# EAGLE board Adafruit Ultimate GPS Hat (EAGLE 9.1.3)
REV: B
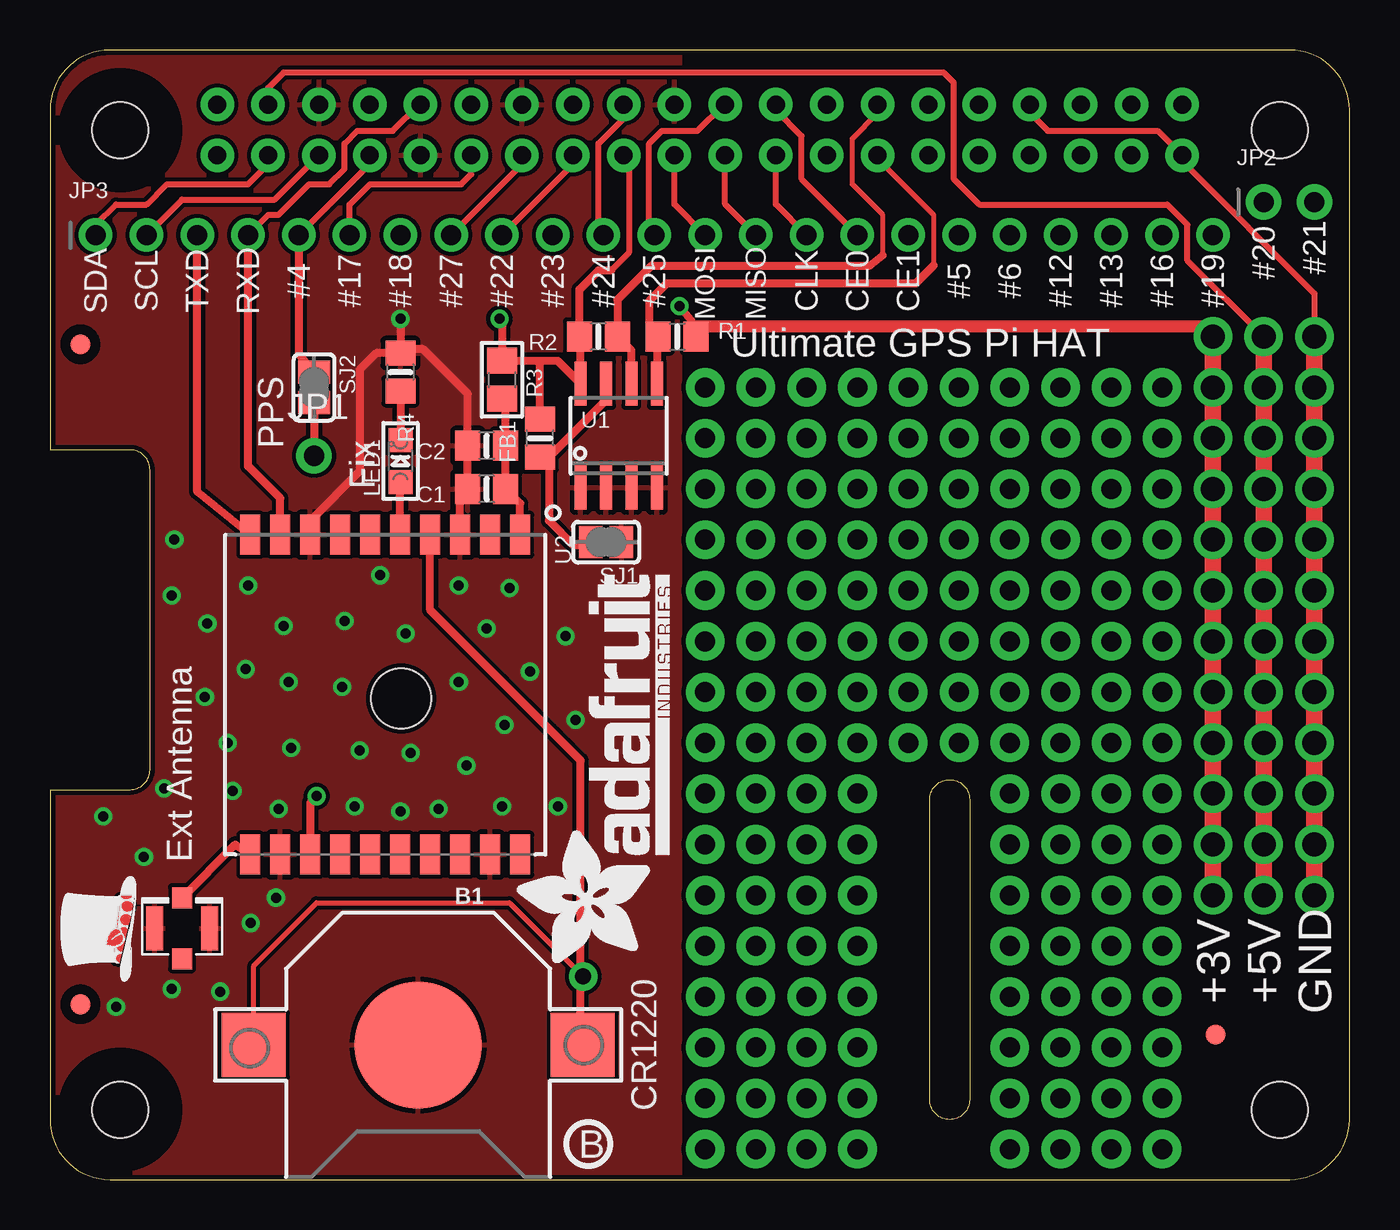
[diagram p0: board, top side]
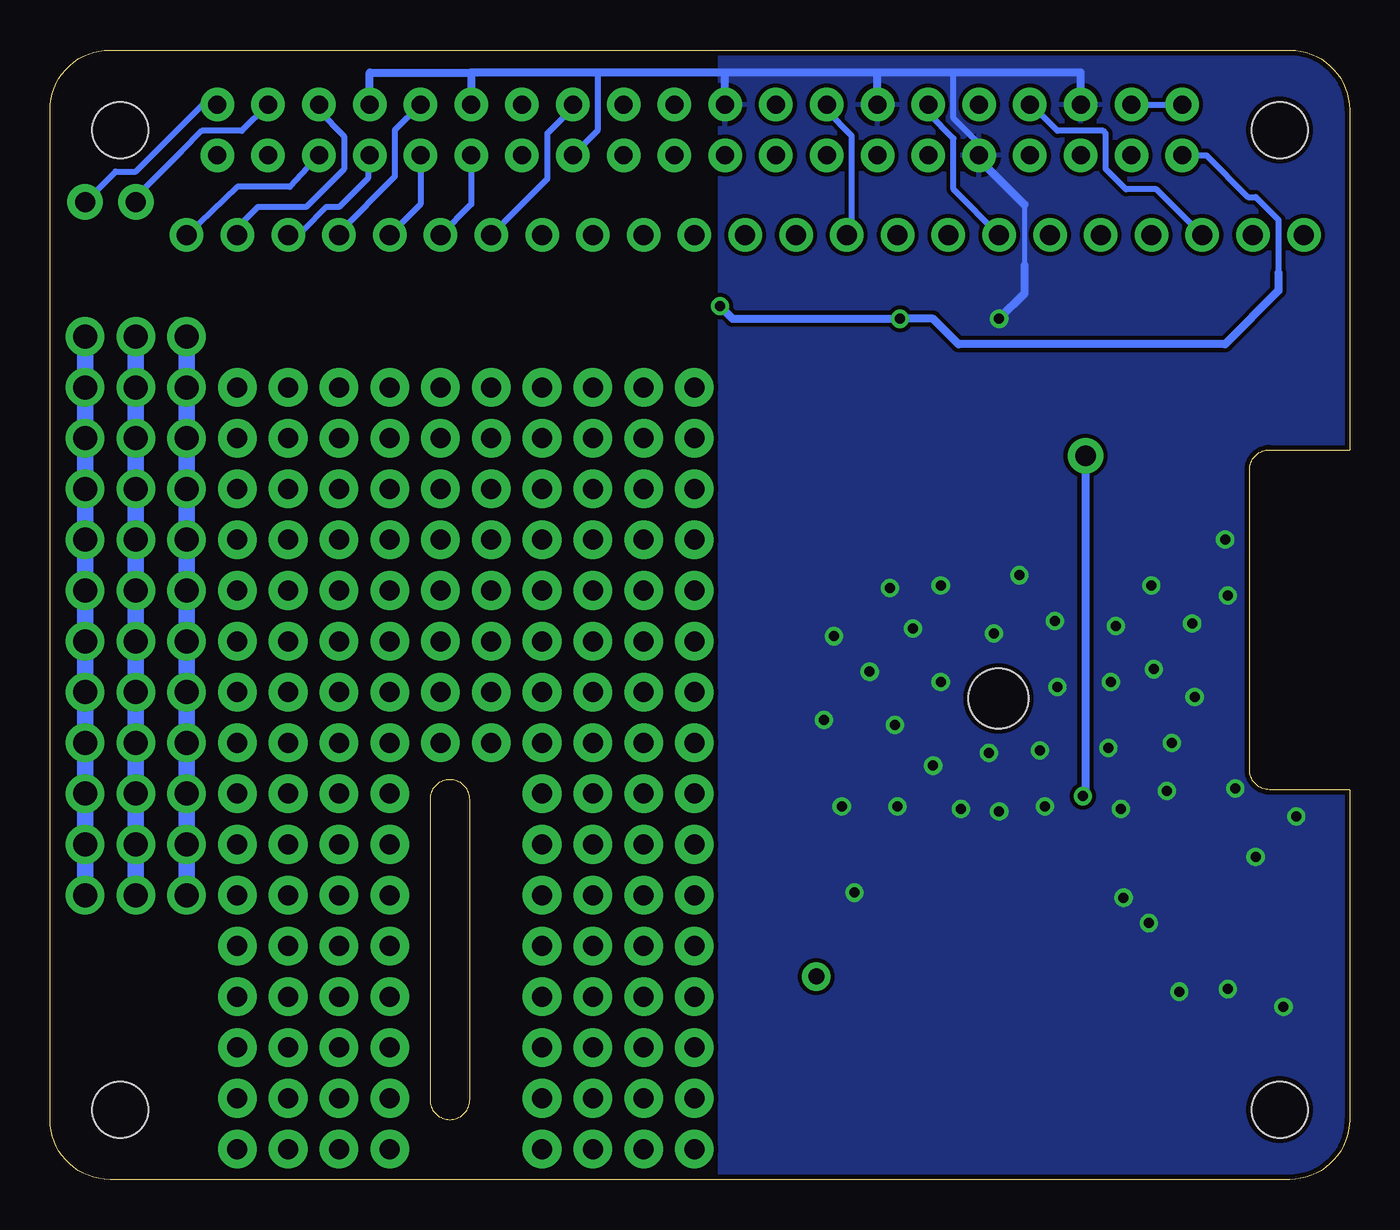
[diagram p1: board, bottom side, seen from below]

Size 65 x 56.5 mm. Coordinates in mm from the lower left corner, seen from the top.
Copper layers (1*16): Top 0.035mm / dielectric 1.5mm / Bottom 0.035mm
Design rules "adafruit": minimum track width 8mil, minimum drill 15.5mil, track to track 8mil, track to pad 8mil, pad to pad 8mil, via to via 8mil, smd to smd 8mil, copper to edge 10mil, drill to drill 8mil, minimum pad ring 10mil, minimum via ring 8mil, stop-mask expansion 2mil, vias tented up to drill 20mil, thermal gap 10mil

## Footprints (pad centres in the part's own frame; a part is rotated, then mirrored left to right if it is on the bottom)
CR1220 = smd 3.2 x 3.2: +$1 -8.225,0; +$2 8.225,0 | smd 6.35 x 6.35: - 0,0
0805-NO = smd 1.24 x 1.5: 1 -0.95,0; 2 0.95,0
0805 = smd 1.3 x 1.5: 1 -0.95,0; 2 0.95,0
FIDUCIAL_1MM = smd 1 x 1: 1 0,0
1X01-CLEANBIG = drill 1.016 pad 1.778: 1 0,0
1X02_ROUND = drill 1 pad 1.778: 1 -1.27,0; 2 1.27,0
1X23_ROUND_70MIL = drill 1 pad 1.676: 1 -27.94,0; 2 -25.4,0; 3 -22.86,0; 4 -20.32,0; 5 -17.78,0; 6 -15.24,0; 7 -12.7,0; 8 -10.16,0; 9 -7.62,0; 10 -5.08,0; 11 -2.54,0; 12 0,0; 13 2.54,0; 14 5.08,0; 15 7.62,0; 16 10.16,0; 17 12.7,0; 18 15.24,0; 19 17.78,0; 20 20.32,0; 21 22.86,0; 22 25.4,0; 23 27.94,0
CHIPLED_0805 = smd 1.2 x 1.2: A 0,-1.05; C 0,1.05
PI_HAT_SLOTS = drill 0.9 pad 1.676: 1 8.37,51.23; 2 8.37,53.77; 3 10.91,51.23; 4 10.91,53.77; 5 13.45,51.23; 6 13.45,53.77; 7 15.99,51.23; 8 15.99,53.77; 9 18.53,51.23; 10 18.53,53.77; 11 21.07,51.23; 12 21.07,53.77; 13 23.61,51.23; 14 23.61,53.77; 15 26.15,51.23; 16 26.15,53.77; 17 28.69,51.23; 18 28.69,53.77; 19 31.23,51.23; 20 31.23,53.77; 21 33.77,51.23; 22 33.77,53.77; 23 36.31,51.23; 24 36.31,53.77; 25 38.85,51.23; 26 38.85,53.77; 27 41.39,51.23; 28 41.39,53.77; 29 43.93,51.23; 30 43.93,53.77; 31 46.47,51.23; 32 46.47,53.77; 33 49.01,51.23; 34 49.01,53.77; 35 51.55,51.23; 36 51.55,53.77; 37 54.09,51.23; 38 54.09,53.77; 39 56.63,51.23; 40 56.63,53.77 | hole 2.8: 3.5,3.5; 3.5,52.5; 61.5,52.5; 61.5,3.5
SOLDERJUMPER_CLOSEDWIRE = smd 1.168 x 1.6: 1 -0.762,0; 2 0.762,0 | smd 0.635 x 0.203: WIRE 0,0
SOIC8_150MIL = smd 0.6 x 2.2: 1 -1.905,-2.6; 2 -0.635,-2.6; 3 0.635,-2.6; 4 1.905,-2.6; 5 1.905,2.6; 6 0.635,2.6; 7 -0.635,2.6; 8 -1.905,2.6
FGPMMOPA6H = smd 2 x 1: P$1 -8,6.75; P$2 -8,5.25; P$3 -8,3.75; P$4 -8,2.25; P$5 -8,0.75; P$6 -8,-0.75; P$7 -8,-2.25; P$8 -8,-3.75; P$9 -8,-5.25; P$10 -8,-6.75; P$11 8,-6.75; P$12 8,-5.25; P$13 8,-3.75; P$14 8,-2.25; P$15 8,-0.75; P$16 8,0.75; P$17 8,2.25; P$18 8,3.75; P$19 8,5.25; P$20 8,6.75 | hole 3: 0.2,0.8
U.FL = smd 2.2 x 0.85: P$1 0,1.375; P$2 0,-1.375 | smd 1.05 x 1: P$3 1.525,0; P$4 -1.525,0

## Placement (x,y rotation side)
B1  CR1220  [CR1220]  18.41,6.73 180 top
C1  0.1uF  [0805-NO]  21.84,34.54 180 top
C2  10uF  [0805-NO]  21.84,36.7 180 top
FB1  Ferrite  [0805]  22.61,40.01 270 top
FID1  FIDUCIAL_1MM  [FIDUCIAL_1MM]  1.52,8.76 0 top
FID2  FIDUCIAL_1MM  [FIDUCIAL_1MM]  1.52,41.78 0 top
FID3  FIDUCIAL_1MM  [FIDUCIAL_1MM]  58.29,7.24 0 top
JP1  [1X01-CLEANBIG]  13.21,36.2 0 top
JP2  [1X02_ROUND]  61.98,48.9 0 top
JP3  [1X23_ROUND_70MIL]  30.23,47.24 0 top
LED1  RED  [CHIPLED_0805]  17.53,35.94 0 top
R1  3.9K  [0805-NO]  31.37,42.16 0 top
R2  3.9K  [0805-NO]  27.43,42.16 180 top
R3  3.9K  [0805-NO]  24.51,37.08 90 top
R4  470  [0805-NO]  17.53,40.39 270 top
RPI1  RASPBERRYPI_BPLUS_HATSLOTS  [PI_HAT_SLOTS]  0,0 0 top
SJ1  WP  [SOLDERJUMPER_CLOSEDWIRE]  27.81,31.88 180 top
SJ2  PPS  [SOLDERJUMPER_CLOSEDWIRE]  13.21,39.62 270 top
U1  CAT24C32  [SOIC8_150MIL]  28.45,37.21 0 top
U2  FGPMMOPA6H  [FGPMMOPA6H]  16.76,24.26 270 top
U$3  [ADAFRUIT_TEXT_20MM]  30.99,10.67 90 top
U$4  [PIHATLOGO]  4.32,9.91 90 top
U$6  [PCBFEAT-REV-056]  26.92,1.78 0 top
U$20  U.FL  [U.FL]  6.6,12.57 90 top

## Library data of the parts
B1 C1 C2 FB1 JP2 JP3 LED1 R1-R4 RPI1 SJ1 SJ2 U1 U2 U$3 U$4 U$6 U$20 = microbuilder
FID1-FID3 = microbuilder; BOM: EXCLUDE
JP1 = adafruit

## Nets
1PPS: JP1.1 SJ2.2 U2.P$13
3.3V: FB1.1 R1.2 R2.2 R3.2 RPI1.1 RPI1.17 U1.8
5.0V: RPI1.2 RPI1.4
EECLK: R2.1 RPI1.28 U1.6
EEDATA: R1.1 RPI1.27 U1.5
FIX: LED1.A U2.P$5
GND: B1.- C1.2 C2.2 R4.1 RPI1.6 RPI1.9 RPI1.14 RPI1.20 RPI1.25 RPI1.30 RPI1.34 RPI1.39 SJ1.1 U1.1 U1.2 U1.3 U1.4 U2.P$3 U2.P$8 U2.P$12 U2.P$19 U$20.P$1 U$20.P$2
GPIO4: JP3.5 RPI1.7 SJ2.1
GPIO5: JP3.18 RPI1.29
GPIO6: JP3.19 RPI1.31
GPIO12: JP3.20 RPI1.32
GPIO13: JP3.21 RPI1.33
GPIO16: JP3.22 RPI1.36
GPIO17: JP3.6 RPI1.11
GPIO18: JP3.7 RPI1.12
GPIO19: JP3.23 RPI1.35
GPIO20: JP2.1 RPI1.38
GPIO21: JP2.2 RPI1.40
GPIO22: JP3.9 RPI1.15
GPIO23: JP3.10 RPI1.16
GPIO24: JP3.11 RPI1.18
GPIO25: JP3.12 RPI1.22
GPIO26: RPI1.37
GPIO27: JP3.8 RPI1.13
N$16: R3.1 SJ1.2 U1.7
N$24: LED1.C R4.2
N$26: U2.P$11 U$20.P$3
RXD: JP3.4 RPI1.10 U2.P$9
SCL: JP3.2 RPI1.5
SDA: JP3.1 RPI1.3
SPI_CE0: JP3.16 RPI1.24
SPI_CE1: JP3.17 RPI1.26
SPI_MISO: JP3.14 RPI1.21
SPI_MOSI: JP3.13 RPI1.19
SPI_SCLK: JP3.15 RPI1.23
TXD: JP3.3 RPI1.8 U2.P$10
VBACKUP: B1.+$1 B1.+$2 U2.P$4
VCC: C1.1 C2.1 FB1.2 U2.P$1

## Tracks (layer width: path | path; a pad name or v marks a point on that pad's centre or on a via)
1PPS  (via drill 0.5)
  Top 0.406: SJ2.2 JP1.1 | v13.34,19.18 13.01,18.86 U2.P$13
  Bottom 0.406: JP1.1 13.21,19.3 v13.34,19.18
3.3V  (via drill 0.5, 1.2 pad 1.93)
  Top 0.305: RPI1.17 28.96,50.96 28.96,46.36 28.07,45.47
  Top 0.406: 24.64,40.95 FB1.1 22.61,42.93 v22.48,43.05 | 24.64,40.95 25.4,40.95 U1.8 26.54,42.23 R2.2 26.48,44.52 27.43,45.47 28.07,45.47 | R1.2 32.07,42.99 v31.5,43.69 | R3.2 24.51,40.83 24.64,40.95
  Top 0.61: v58.17,42.16 57.66,42.67 32,42.67 32.07,42.61 R1.2
  Top 0.813: v58.17,42.16 v58.17,14.22
  Bottom 0.305: RPI1.1 7.16,51.23 5.08,49.15 4.7,49.15 3.56,48.01 3.56,45.34
  Bottom 0.406: 3.56,45.34 3.56,44.45 6.22,41.78 19.56,41.78 20.83,43.05 v22.48,43.05 30.86,43.05 v31.5,43.69
  Bottom 0.813: v58.17,14.22 v58.17,16.76 v58.17,19.3 v58.17,21.84 v58.17,24.38 v58.17,26.92 v58.17,29.46 v58.17,32 v58.17,34.54 v58.17,37.08 v58.17,39.62 v58.17,42.16
5.0V  (via drill 1.2 pad 1.93)
  Top 0.305: RPI1.4 10.91,54.6 11.68,55.37 44.7,55.37 45.21,54.86 45.21,50.04 46.48,48.77 55.88,48.77 56.9,47.75 56.9,45.97 v60.71,42.16
  Top 0.813: v60.71,42.16 60.71,13.97
  Bottom 0.305: RPI1.4 RPI1.2
  Bottom 0.813: v60.71,14.22 v60.71,16.76 v60.71,19.3 v60.71,21.84 v60.71,24.38 v60.71,26.92 v60.71,29.46 v60.71,32 v60.71,34.54 v60.71,37.08 v60.71,39.62 v60.71,42.16
EECLK
  Top 0.254: 41.66,46.23 41.66,48.26 40.13,49.78 40.13,52.07 41.39,53.33 RPI1.28
  Top 0.406: 41.66,46.23 41.02,45.72 30.1,45.72 28.38,44 R2.1 29.08,41.46 U1.6
EEDATA
  Top 0.254: RPI1.27 41.39,51.07 44.2,48.26 44.2,45.72
  Top 0.406: 44.2,45.72 43.31,44.83 30.86,44.83 29.97,43.94 29.97,42.16 30.35,42.16 | 30.35,42.16 U1.5 | R1.1 30.35,42.16
FIX
  Top 0.406: U2.P$5 17.51,34.88 LED1.A
GND  (via drill 0.5, 1.2 pad 1.93)
  Top 0.305: RPI1.34 49.01,53.35 49.91,52.45 55.41,52.45 RPI1.39 56.63,50.94 63.25,44.32 v63.25,42.16
  Top 0.406: U2.P$3 20.51,34.54 C1.2 C2.2 20.89,39.3 18.67,41.53 17.72,41.53 R4.1 | v17.53,43.05 R4.1 | R4.1 16.32,41.34 15.49,40.51 15.49,35.43 13.08,33.02 13.08,31.82 U2.P$8
  Top 0.813: v63.25,42.16 v63.25,14.22
  Bottom 0.254: 16.26,48.77 16.26,45.72
  Bottom 0.305: 19.94,55.37 19.81,55.25 19.81,53.09 18.53,51.8 RPI1.9 18.53,51.04 | RPI1.25 37.59,52.49 37.59,55.37
  Bottom 0.406: RPI1.34 49.01,55.37 43.94,55.37 | 43.94,55.37 43.94,53.77 RPI1.30 | RPI1.20 31.23,55.37 | 31.23,55.37 37.59,55.37 43.94,55.37 | RPI1.14 23.61,55.37 | 23.61,55.37 31.23,55.37 | RPI1.6 13.45,55.37 19.94,55.37 23.61,55.37 | 18.53,51.04 16.26,48.77 | 16.26,45.72 16.26,44.32 v17.53,43.05
  Bottom 0.813: v63.25,14.22 v63.25,16.76 v63.25,19.3 v63.25,21.84 v63.25,24.38 v63.25,26.92 v63.25,29.46 v63.25,32 v63.25,34.54 v63.25,37.08 v63.25,39.62 v63.25,42.16
  other vias: 11.43,18.54 9.14,19.43 8.89,21.84 12.07,21.59 11.94,24.89 11.68,27.69 9.78,25.53 9.91,29.72 6.22,32 6.1,29.21 5.71,19.56 7.75,24.13 7.87,27.81 2.67,18.16 4.7,16.13 6.1,9.53 3.3,8.64 8.51,9.4 10.03,12.83 15.24,18.67 15.49,21.46 14.61,24.64 14.73,27.94 16.51,30.23 17.78,27.3 20.45,29.72 22.99,29.59 21.84,27.56 24,25.4 26.29,22.99 25.4,18.67 22.61,18.67 22.73,22.73 20.45,24.89 20.83,20.7 19.43,18.54 18.03,21.34 17.53,18.41 25.78,27.18 11.3,14.1 24.76,14.35
  pour Top: -0.25,56.52 31.5,56.52 31.5,0 -0.25,0
  pour Bottom: -0.25,56.52 31.5,56.52 31.5,0 -0.25,0
GPIO4
  Top 0.305: JP3.5 15.99,50.79 RPI1.7
  Top 0.406: JP3.5 12.45,41.27 SJ2.1
GPIO5
  Bottom 0.305: RPI1.29 43.93,48.78 JP3.18
GPIO6
  Bottom 0.305: RPI1.31 46.47,48.78 JP3.19
GPIO12
  Bottom 0.305: RPI1.32 47.75,52.49 47.75,50.16 50.55,47.37 JP3.20
GPIO13
  Bottom 0.305: RPI1.33 49.1,51.23 49.1,50.09 50.55,48.64 51.18,48.64 52.32,47.5 52.83,47.5 JP3.21
GPIO16
  Bottom 0.305: RPI1.36 51.55,53.45 50.29,52.2 50.29,50.55 52.2,48.64 54.61,48.64 55.63,47.62 JP3.22
GPIO17
  Top 0.305: JP3.6 14.99,48.77 16,49.78 20.57,49.78 21.07,50.28 RPI1.11
GPIO18
  Bottom 0.305: JP3.7 19.81,49.53 19.81,52.07 21.07,53.33 RPI1.12
GPIO19
  Bottom 0.305: RPI1.35 53,49.66 55.63,49.66 JP3.23
GPIO20
  Bottom 0.305: RPI1.38 55.41,52.45 57.4,52.45 58.42,51.44 60.71,49.15 JP2.1
GPIO21
  Bottom 0.305: RPI1.40 56.68,53.72 57.4,53.72 60.71,50.42 61.72,50.42 JP2.2
GPIO22
  Top 0.305: JP3.9 26.15,50.79 RPI1.15
GPIO23
  Bottom 0.305: JP3.10 24.89,47.5 24.89,52.2 26.15,53.45 RPI1.16
GPIO24
  Top 0.305: JP3.11 27.43,47.5 27.43,51.82 28.69,53.07 RPI1.18
GPIO25
  Top 0.305: JP3.12 29.97,47.5 29.97,51.82 30.61,52.45 32.39,52.45 33.7,53.77 RPI1.22
GPIO27
  Top 0.305: JP3.8 23.61,50.79 RPI1.13
N$1  (via drill 1 pad 1.93)
  other vias: 55.63,39.62
N$2  (via drill 1 pad 1.93)
  other vias: 55.63,37.08
N$3  (via drill 1 pad 1.93)
  other vias: 55.63,34.54
N$4  (via drill 1 pad 1.93)
  other vias: 53.09,34.54
N$5  (via drill 1 pad 1.93)
  other vias: 53.09,37.08
N$6  (via drill 1 pad 1.93)
  other vias: 53.09,39.62
N$7  (via drill 1 pad 1.93)
  other vias: 48.01,39.62
N$8  (via drill 1 pad 1.93)
  other vias: 50.55,34.54
N$9  (via drill 1 pad 1.93)
  other vias: 48.01,37.08
N$10  (via drill 1 pad 1.93)
  other vias: 48.01,34.54
N$11  (via drill 1 pad 1.93)
  other vias: 50.55,37.08
N$12  (via drill 1 pad 1.93)
  other vias: 50.55,39.62
N$13  (via drill 1 pad 1.93)
  other vias: 45.47,39.62
N$14  (via drill 1 pad 1.93)
  other vias: 45.47,37.08
N$15  (via drill 1 pad 1.93)
  other vias: 45.47,34.54
N$16
  Top 0.406: R3.1 24.96,36.13 | 24.96,36.13 27.81,38.99 U1.7 | 24.96,36.13 24.96,32.95 26.16,31.75 26.92,31.75 SJ1.2
N$17  (via drill 1 pad 1.93)
  other vias: 42.93,34.54
N$18  (via drill 1 pad 1.93)
  other vias: 42.93,37.08
N$19  (via drill 1 pad 1.93)
  other vias: 42.93,39.62
N$20  (via drill 1 pad 1.93)
  other vias: 40.39,39.62
N$21  (via drill 1 pad 1.93)
  other vias: 40.39,37.08
N$22  (via drill 1 pad 1.93)
  other vias: 40.39,34.54
N$23  (via drill 1 pad 1.93)
  other vias: 37.85,34.54
N$24
  Top 0.406: R4.2 LED1.C
N$25  (via drill 1 pad 1.93)
  other vias: 37.85,37.08
N$26
  Top 0.406: U$20.P$3 9.26,16.76 U2.P$11
N$27  (via drill 1 pad 1.93)
  other vias: 37.85,39.62
N$28  (via drill 1 pad 1.93)
  other vias: 35.31,39.62
N$29  (via drill 1 pad 1.93)
  other vias: 35.31,34.54
N$30  (via drill 1 pad 1.93)
  other vias: 35.31,37.08
N$31  (via drill 1 pad 1.93)
  other vias: 32.77,39.62
N$32  (via drill 1 pad 1.93)
  other vias: 32.77,37.08
N$33  (via drill 1 pad 1.93)
  other vias: 32.77,34.54
N$34  (via drill 1 pad 1.93)
  other vias: 32.77,32
N$35  (via drill 1 pad 1.93)
  other vias: 35.31,32
N$36  (via drill 1 pad 1.93)
  other vias: 37.85,32
N$37  (via drill 1 pad 1.93)
  other vias: 40.39,32
N$38  (via drill 1 pad 1.93)
  other vias: 45.47,32
N$39  (via drill 1 pad 1.93)
  other vias: 42.93,32
N$40  (via drill 1 pad 1.93)
  other vias: 50.55,32
N$41  (via drill 1 pad 1.93)
  other vias: 53.09,32
N$42  (via drill 1 pad 1.93)
  other vias: 55.63,32
N$43  (via drill 1 pad 1.93)
  other vias: 48.01,32
N$44  (via drill 1 pad 1.93)
  other vias: 32.77,29.46
N$45  (via drill 1 pad 1.93)
  other vias: 32.77,26.92
N$46  (via drill 1 pad 1.93)
  other vias: 32.77,24.38
N$47  (via drill 1 pad 1.93)
  other vias: 32.77,21.84
N$48  (via drill 1 pad 1.93)
  other vias: 32.77,16.76
N$49  (via drill 1 pad 1.93)
  other vias: 32.77,19.3
N$50  (via drill 1 pad 1.93)
  other vias: 32.77,14.22
N$51  (via drill 1 pad 1.93)
  other vias: 32.77,11.68
N$52  (via drill 1 pad 1.93)
  other vias: 32.77,9.14
N$53  (via drill 1 pad 1.93)
  other vias: 32.77,6.6
N$54  (via drill 1 pad 1.93)
  other vias: 32.77,4.06
N$55  (via drill 1 pad 1.93)
  other vias: 32.77,1.52
N$56  (via drill 1 pad 1.93)
  other vias: 35.31,1.52
N$57  (via drill 1 pad 1.93)
  other vias: 35.31,4.06
N$58  (via drill 1 pad 1.93)
  other vias: 37.85,6.6
N$59  (via drill 1 pad 1.93)
  other vias: 35.31,6.6
N$60  (via drill 1 pad 1.93)
  other vias: 35.31,9.14
N$61  (via drill 1 pad 1.93)
  other vias: 35.31,11.68
N$62  (via drill 1 pad 1.93)
  other vias: 35.31,14.22
N$63  (via drill 1 pad 1.93)
  other vias: 35.31,16.76
N$64  (via drill 1 pad 1.93)
  other vias: 35.31,19.3
N$65  (via drill 1 pad 1.93)
  other vias: 35.31,21.84
N$66  (via drill 1 pad 1.93)
  other vias: 35.31,24.38
N$67  (via drill 1 pad 1.93)
  other vias: 35.31,26.92
N$68  (via drill 1 pad 1.93)
  other vias: 35.31,29.46
N$69  (via drill 1 pad 1.93)
  other vias: 37.85,29.46
N$70  (via drill 1 pad 1.93)
  other vias: 37.85,24.38
N$71  (via drill 1 pad 1.93)
  other vias: 37.85,26.92
N$72  (via drill 1 pad 1.93)
  other vias: 37.85,21.84
N$73  (via drill 1 pad 1.93)
  other vias: 37.85,19.3
N$74  (via drill 1 pad 1.93)
  other vias: 37.85,16.76
N$75  (via drill 1 pad 1.93)
  other vias: 37.85,14.22
N$76  (via drill 1 pad 1.93)
  other vias: 37.85,11.68
N$77  (via drill 1 pad 1.93)
  other vias: 37.85,9.14
N$78  (via drill 1 pad 1.93)
  other vias: 37.85,4.06
N$79  (via drill 1 pad 1.93)
  other vias: 37.85,1.52
N$80  (via drill 1 pad 1.93)
  other vias: 40.39,1.52
N$81  (via drill 1 pad 1.93)
  other vias: 40.39,4.06
N$82  (via drill 1 pad 1.93)
  other vias: 40.39,6.6
N$83  (via drill 1 pad 1.93)
  other vias: 40.39,9.14
N$84  (via drill 1 pad 1.93)
  other vias: 40.39,11.68
N$85  (via drill 1 pad 1.93)
  other vias: 40.39,14.22
N$86  (via drill 1 pad 1.93)
  other vias: 40.39,16.76
N$87  (via drill 1 pad 1.93)
  other vias: 40.39,21.84
N$88  (via drill 1 pad 1.93)
  other vias: 40.39,24.38
N$89  (via drill 1 pad 1.93)
  other vias: 40.39,26.92
N$90  (via drill 1 pad 1.93)
  other vias: 40.39,29.46
N$91  (via drill 1 pad 1.93)
  other vias: 42.93,29.46
N$92  (via drill 1 pad 1.93)
  other vias: 42.93,26.92
N$93  (via drill 1 pad 1.93)
  other vias: 42.93,24.38
N$94  (via drill 1 pad 1.93)
  other vias: 42.93,21.84
N$95  (via drill 1 pad 1.93)
  other vias: 40.39,19.3
N$96  (via drill 1 pad 1.93)
  other vias: 48.01,1.52
N$97  (via drill 1 pad 1.93)
  other vias: 48.01,6.6
N$98  (via drill 1 pad 1.93)
  other vias: 48.01,4.06
N$99  (via drill 1 pad 1.93)
  other vias: 48.01,9.14
N$100  (via drill 1 pad 1.93)
  other vias: 48.01,11.68
N$101  (via drill 1 pad 1.93)
  other vias: 48.01,14.22
N$102  (via drill 1 pad 1.93)
  other vias: 48.01,19.3
N$103  (via drill 1 pad 1.93)
  other vias: 48.01,21.84
N$104  (via drill 1 pad 1.93)
  other vias: 48.01,24.38
N$105  (via drill 1 pad 1.93)
  other vias: 48.01,26.92
N$106  (via drill 1 pad 1.93)
  other vias: 48.01,29.46
N$107  (via drill 1 pad 1.93)
  other vias: 45.47,29.46
N$108  (via drill 1 pad 1.93)
  other vias: 45.47,26.92
N$109  (via drill 1 pad 1.93)
  other vias: 45.47,24.38
N$110  (via drill 1 pad 1.93)
  other vias: 45.47,21.84
N$111  (via drill 1 pad 1.93)
  other vias: 50.55,29.46
N$112  (via drill 1 pad 1.93)
  other vias: 53.09,29.46
N$113  (via drill 1 pad 1.93)
  other vias: 55.63,29.46
N$114  (via drill 1 pad 1.93)
  other vias: 55.63,26.92
N$115  (via drill 1 pad 1.93)
  other vias: 53.09,26.92
N$116  (via drill 1 pad 1.93)
  other vias: 50.55,26.92
N$117  (via drill 1 pad 1.93)
  other vias: 50.55,24.38
N$118  (via drill 1 pad 1.93)
  other vias: 55.63,24.38
N$119  (via drill 1 pad 1.93)
  other vias: 53.09,24.38
N$120  (via drill 1 pad 1.93)
  other vias: 53.09,21.84
N$121  (via drill 1 pad 1.93)
  other vias: 50.55,21.84
N$122  (via drill 1 pad 1.93)
  other vias: 50.55,19.3
N$123  (via drill 1 pad 1.93)
  other vias: 53.09,19.3
N$124  (via drill 1 pad 1.93)
  other vias: 55.63,19.3
N$125  (via drill 1 pad 1.93)
  other vias: 55.63,21.84
N$126  (via drill 1 pad 1.93)
  other vias: 55.63,16.76
N$127  (via drill 1 pad 1.93)
  other vias: 53.09,16.76
N$128  (via drill 1 pad 1.93)
  other vias: 50.55,16.76
N$129  (via drill 1 pad 1.93)
  other vias: 48.01,16.76
N$130  (via drill 1 pad 1.93)
  other vias: 50.55,14.22
N$131  (via drill 1 pad 1.93)
  other vias: 53.09,14.22
N$132  (via drill 1 pad 1.93)
  other vias: 55.63,14.22
N$133  (via drill 1 pad 1.93)
  other vias: 55.63,11.68
N$134  (via drill 1 pad 1.93)
  other vias: 50.55,11.68
N$135  (via drill 1 pad 1.93)
  other vias: 50.55,9.14
N$136  (via drill 1 pad 1.93)
  other vias: 50.55,6.6
N$137  (via drill 1 pad 1.93)
  other vias: 50.55,4.06
N$138  (via drill 1 pad 1.93)
  other vias: 50.55,1.52
N$139  (via drill 1 pad 1.93)
  other vias: 53.09,1.52
N$140  (via drill 1 pad 1.93)
  other vias: 53.09,4.06
N$141  (via drill 1 pad 1.93)
  other vias: 53.09,6.6
N$142  (via drill 1 pad 1.93)
  other vias: 53.09,11.68
N$143  (via drill 1 pad 1.93)
  other vias: 55.63,9.14
N$144  (via drill 1 pad 1.93)
  other vias: 53.09,9.14
N$145  (via drill 1 pad 1.93)
  other vias: 55.63,6.6
N$146  (via drill 1 pad 1.93)
  other vias: 55.63,4.06
N$147  (via drill 1 pad 1.93)
  other vias: 55.63,1.52
RXD
  Top 0.305: JP3.4 10.92,48.26 11.43,48.26 12.95,49.78 13.97,49.78 14.73,50.55 14.73,51.82 15.37,52.45 17.14,52.45 18.46,53.77 RPI1.10
  Top 0.406: U2.P$9 11.51,34.08 9.91,35.69 JP3.4
SCL
  Top 0.305: JP3.2 6.6,49.02 11.24,49.02 RPI1.5
SDA
  Top 0.305: JP3.1 2.29,47.75 3.3,48.77 4.83,48.77 5.84,49.78 9.91,49.78 10.91,50.79 RPI1.3
SPI_CE0
  Top 0.305: JP3.16 37.59,50.04 37.59,52.2 36.31,53.48 RPI1.24
SPI_CE1
  Bottom 0.305: RPI1.26 38.85,53.61 40.13,52.32 40.13,50.04 JP3.17
SPI_MISO
  Top 0.305: JP3.14 33.77,48.78 RPI1.21
SPI_MOSI
  Top 0.305: JP3.13 31.23,48.78 RPI1.19
SPI_SCLK
  Top 0.305: JP3.15 36.31,48.78 RPI1.23
TXD
  Top 0.406: U2.P$10 7.37,34.41 JP3.3
  Bottom 0.305: JP3.3 9.65,49.53 11.18,49.53 12.19,50.55 12.19,52.32 12.32,52.45 14.61,52.45 15.92,53.77 RPI1.8
VBACKUP  (via drill 0.8 pad 1.42)
  Top 0.254: B1.+$2 10.19,10.7 13.34,13.84 22.99,13.84 v26.67,10.16
  Top 0.406: 26.54,10.16 26.54,7.38 26.64,7.46 26.64,7.34 B1.+$1 | U2.P$4 19.01,28.48 26.54,20.95 26.54,10.16 | 26.54,10.16 v26.67,10.16
VCC
  Top 0.406: U2.P$1 23.51,33.82 C1.1 C2.1 22.79,38.87 FB1.2

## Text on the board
tPlace: #21 | #20 | SDA | SCL | TXD | RXD | #4 | #17 | #18 | #27 | #22 | #23 | #24 | #25 | MOSI | MISO | CLK | CE0 | CE1 | #5 | #6 | #12 | #13 | #16 | #19 | Ultimate GPS Pi HAT | PPS | Fix | Ext Antenna | +3V | +5V | GND | CR1220

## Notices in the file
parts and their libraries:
microbuilder: This work is placed in the public domain, and may be freely used for commercial and non-commercial work with the following conditions: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
